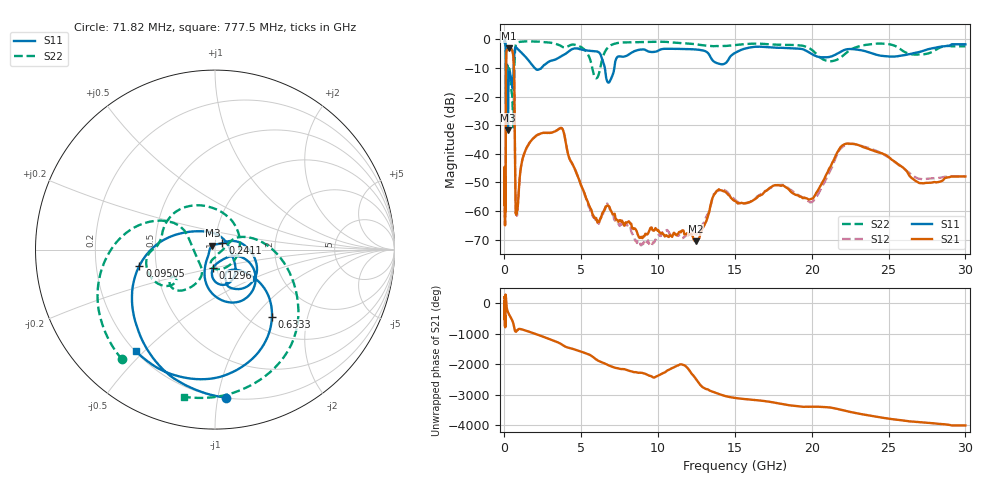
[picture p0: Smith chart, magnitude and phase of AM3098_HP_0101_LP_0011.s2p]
! Date/Time: Thu, Feb 28, 2019 8:36 AM
! Network Analyzer: Agilent Technologies E8364B Rev: A.07.50.67
! Sweep from 0.010 to 30.000 GHz, 1601 Points, Sweep Type: LOG
! Power Supply: 5.023 V, 0.002 A
# Hz S DB R 50
!freq MagS11 AngS11 MagS21 AngS21 MagS12 AngS12 MagS22 AngS22
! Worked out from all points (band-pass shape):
!   1601 points, 10 MHz to 30 GHz, reference 50 ohm
!   highest |S21| = -3.06 dB at 267.8 MHz (marker M1); lowest = -70.7 dB at 12.43 GHz (marker M2)
!   |S21| within 3 dB of the highest: 113.4 MHz to 576.8 MHz (463.4 MHz wide, 134 % of centre)
!   lowest |S11| = -31.8 dB at 230.5 MHz (marker M3), VSWR 1.05, Z = 48.6 + j2.09 ohm
!   |S11| at or under -10 dB: 176.1 MHz to 598.4 MHz (422.3 MHz wide, 109 % of centre); 1.977 GHz to 2.398 GHz (421.5 MHz wide, 19.3 % of centre); 6.532 GHz to 7.148 GHz (616.5 MHz wide, 9.01 % of centre)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
!   |S22| runs from -30.8 to -0.5 dB; largest |S21 - S12| = 0.011
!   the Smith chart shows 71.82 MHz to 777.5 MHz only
!   S11 on the Smith chart (normalised r, x): 71.82 MHz: 0.20, -1.05; 95.05 MHz: 0.40, -0.09; 129.6 MHz: 0.96, -0.20; 241.1 MHz: 1.08, +0.08; 633.3 MHz: 1.25, -1.24; 777.5 MHz: 0.20, -0.47
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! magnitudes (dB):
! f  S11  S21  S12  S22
! 10 MHz  -0.4  -45.6  -45.1  -0.5
! 38.04 MHz  -0.5  -62.9  -60.9  -0.8
! 71.82 MHz  -1.7  -53.5  -52.9  -1.9
! 95.05 MHz  -7.3  -22.5  -22.5  -8.6
! 129.6 MHz  -19.8  -4.5  -4.5  -10.7
! 144.7 MHz  -16.6  -3.8  -3.8  -10.9
! 185.8 MHz  -11.0  -3.6  -3.6  -8.1
! 230.5 MHz  -31.8  -3.2  -3.1  -9.8
! 241.1 MHz  -25.2  -3.1  -3.1  -10.0
! 267.8 MHz  -15.1  -3.1  -3.0  -10.3
! 550.5 MHz  -15.9  -5.0  -4.9  -27.1
! 633.3 MHz  -6.2  -13.6  -13.5  -12.2
! 717.7 MHz  -2.7  -55.9  -54.5  -2.4
! 777.5 MHz  -2.9  -60.4  -61.2  -1.5
! 2.084 GHz  -10.5  -33.6  -33.7  -0.8
! 3.723 GHz  -5.8  -31.0  -31.0  -2.4
! 7.926 GHz  -5.8  -64.1  -64.5  -1.0
! 12.43 GHz  -3.5  -70.7  -68.1  -1.6
! 14.02 GHz  -8.6  -52.7  -52.6  -2.3
! 19.9 GHz  -4.8  -55.9  -57.0  -3.3
! 22.56 GHz  -3.3  -36.5  -36.5  -3.5
! 30 GHz  -1.7  -47.9  -47.9  -2.4
